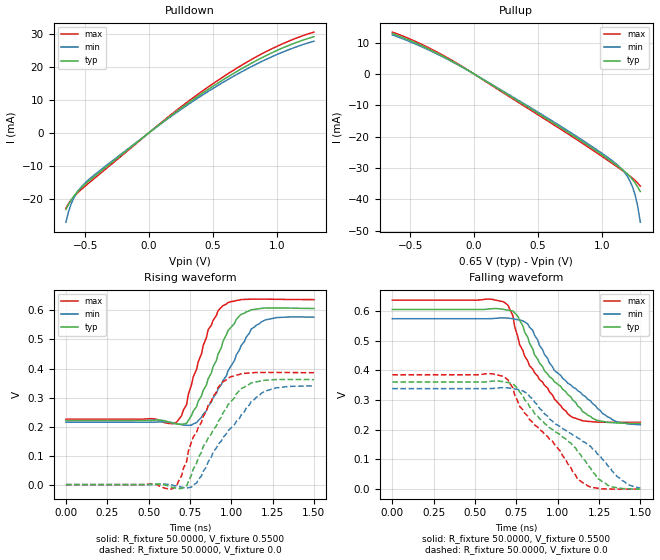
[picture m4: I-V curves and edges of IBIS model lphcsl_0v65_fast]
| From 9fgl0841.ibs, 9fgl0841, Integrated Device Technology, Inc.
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[Model]   lphcsl_0v65_fast
Model_type Output
Polarity   Non-Inverting
Enable   Active-High
Vmeas =  0.4000V
Cref =   2.0000pF
Rref =   0.0
Vref =   0.4000V
C_comp   1.1000pF   1.0000pF   1.2000pF
[Temperature Range]   25.0000   85.0000   -40.0000
[Voltage Range]   0.6500V   0.6200V   0.6800V
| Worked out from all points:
|   slope of the pulldown table from 0 to 0.098 V, typ, clamps not added: 32.8 ohm
|   slope of the pullup table from 0 to 0.098 V, typ, clamps not added: 40 ohm
|   rising waveform, R_fixture 50.0000, V_fixture 0.5500: 20-80 % time 168ps typ, 206ps min, 144ps max; typ from 0.221 V to 0.607 V
|   rising waveform, R_fixture 50.0000, V_fixture 0.0: 20-80 % time 214ps typ, 251ps min, 168ps max; typ from 0 V to 0.362 V
|   falling waveform, R_fixture 50.0000, V_fixture 0.5500: 20-80 % time 294ps typ, 332ps min, 239ps max; typ from 0.606 V to 0.222 V
|   falling waveform, R_fixture 50.0000, V_fixture 0.0: 20-80 % time 376ps typ, 429ps min, 326ps max; typ from 0.361 V to 0 V
[Pulldown]
|Voltage   I(typ)   I(min)   I(max)
-650mV    -23.23mA   -27.08mA   -22.85mA
-630mV    -21.73mA   -23.92mA   -21.53mA
-610mV    -20.42mA   -21.63mA   -20.41mA
-590mV    -19.28mA   -19.88mA   -19.45mA
-550mV    -17.42mA   -17.37mA   -17.87mA
-510mV    -15.92mA   -15.58mA   -16.5mA
-350mV    -10.82mA   -10.4mA    -11.34mA
130mV     3.938mA    3.75mA     4.173mA
450mV     12.8mA     12.19mA    13.51mA
770mV     20.38mA    19.39mA    21.48mA
1.03V     25.42mA    24.16mA    26.67mA
1.29V     29.08mA    27.71mA    30.47mA
[Pullup]
|Voltage   I(typ)   I(min)   I(max)
-640mV    12.9mA     12.48mA    13.37mA
-340mV    7.668mA    7.369mA    8.057mA
-40mV     988uA      943.5uA    1.052mA
700mV     -17.66mA   -17.23mA   -18.19mA
1.08V     -28.05mA   -27.62mA   -28.49mA
1.16V     -30.49mA   -30.54mA   -30.78mA
1.2V      -31.91mA   -32.71mA   -31.96mA
1.22V     -32.74mA   -34.19mA   -32.58mA
1.24V     -33.69mA   -36.08mA   -33.24mA
1.26V     -34.78mA   -38.62mA   -33.96mA
1.28V     -36.03mA   -42.17mA   -34.78mA
1.3V      -37.46mA   -47.25mA   -35.74mA
[Ramp]
| variable   typ   min   max
dV/dt_r  0.2171/0.2129n   0.2039/0.2456n   0.2314/0.1862n
dV/dt_f  0.2322/0.2706n   0.2162/0.3099n   0.2487/0.2338n
R_load = 50.0000
[Rising Waveform]
R_fixture= 50.0000
V_fixture= 0.5500
V_fixture_min= 0.5200
V_fixture_max= 0.5800
|time   V(typ)   V(min)   V(max)
0s        221mV      214.9mV    225.3mV
650ps     210.5mV    212.1mV    210.1mV
730ps     211.4mV    204.5mV    276.1mV
790ps     268.6mV    213.4mV    396.8mV
860ps     364.5mV    269.7mV    533.4mV
950ps     494mV      359.2mV    616.5mV
1.05ns    581.6mV    464.5mV    635.9mV
1.15ns    604.7mV    548.6mV    639.1mV
1.27ns    608.6mV    575.2mV    638.3mV
1.5ns     606.8mV    576.9mV    637.3mV
[Rising Waveform]
R_fixture= 50.0000
V_fixture= 0.0
V_fixture_min= 0.0
V_fixture_max= 0.0
|time   V(typ)   V(min)   V(max)
0s        0V         0V         0V
640ps     -8.434mV   -704uV     -15.02mV
700ps     -13.35mV   -8.846mV   31.11mV
730ps     -5.209mV   -11.48mV   79.09mV
760ps     34.44mV    -8.318mV   147.9mV
790ps     73.04mV    5.508mV    180.3mV
950ps     247.4mV    162.6mV    354.6mV
1.06ns    330.8mV    239.9mV    381.8mV
1.2ns     359.3mV    320.7mV    386.4mV
1.5ns     361.8mV    339.9mV    385.6mV
[Falling Waveform]
R_fixture= 50.0000
V_fixture= 0.5500
V_fixture_min= 0.5200
V_fixture_max= 0.5800
|time   V(typ)   V(min)   V(max)
0s        605.5mV    574.4mV    637mV
610ps     608.4mV    574.9mV    639.2mV
730ps     600.1mV    574.5mV    584.1mV
770ps     569.5mV    570.1mV    487.1mV
830ps     491.6mV    545.6mV    416.2mV
920ps     399.1mV    454.6mV    350.4mV
1.06ns    319.5mV    357.6mV    254.3mV
1.23ns    233.7mV    280.6mV    226.2mV
1.36ns    223mV      226.1mV    225.3mV
1.5ns     221.5mV    216.9mV    225.3mV
[Falling Waveform]
R_fixture= 50.0000
V_fixture= 0.0
V_fixture_min= 0.0
V_fixture_max= 0.0
|time   V(typ)   V(min)   V(max)
0s        361mV      338.8mV    385.4mV
610ps     364mV      339.3mV    388.2mV
680ps     360.8mV    341.6mV    377mV
730ps     355.5mV    339.4mV    341.2mV
770ps     327.7mV    334.4mV    279.2mV
970ps     200.9mV    228.4mV    160.8mV
1.12ns    126.5mV    172.8mV    33.06mV
1.3ns     13.89mV    80.88mV    422.7uV
1.42ns    1.232mV    16.25mV    -179.8uV
1.5ns     169.3uV    3.586mV    -100uV
